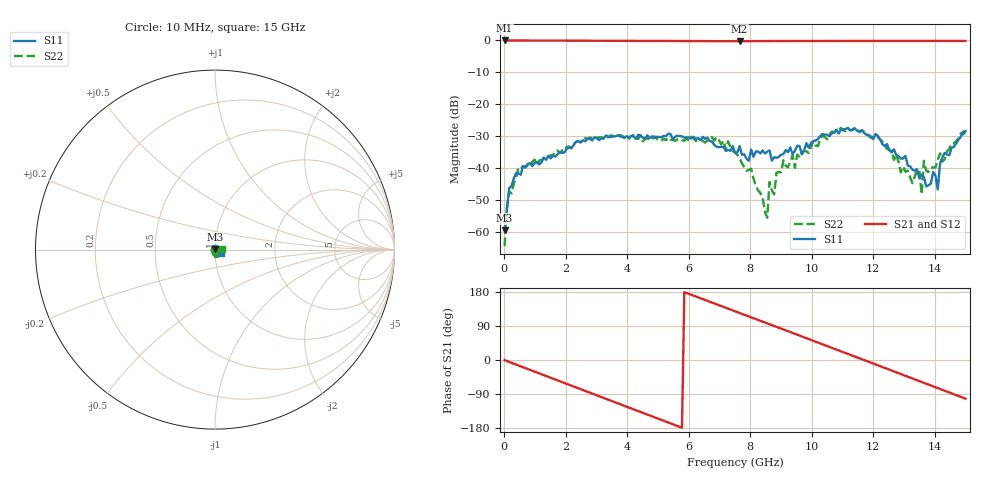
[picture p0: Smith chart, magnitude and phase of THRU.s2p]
#  HZ  S  DB  R  50.00
! Rohde & Schwarz Vector Network Analyzer
! Rohde-Schwarz,ZNB3044-4Port,1351505044101548,4.21
! Created: UTC 8/5/2026, 7:45:01 PM
! freq[Hz]  db:S11  ang:S11  db:S21  ang:S21  db:S12  ang:S12  db:S22  ang:S22
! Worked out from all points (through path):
!   201 points, 10 MHz to 15 GHz, reference 50 ohm
!   highest |S21| = 0.00 dB at 10 MHz (marker M1); lowest = -0.2 dB at 7.655 GHz (marker M2)
!   group delay of S21, straight-line fit = 85.4 ps
!   lowest |S11| = -59.6 dB at 10 MHz (marker M3), VSWR 1.00, Z = 50.1 + j0.0742 ohm
!   |S11| at or under -10 dB: start of sweep to end of sweep
!   |S22| runs from -64.6 to -27.4 dB; largest |S21 - S12| = 0.0051
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1e7  -59.61 45.1  -0.00 -0.4  -0.00 -0.3  -64.59 24.4
1.599e8  -46.34 44.9  -0.01 -5.1  -0.02 -5.1  -47.37 68.3
4.597e8  -41.70 35.1  -0.03 -14.5  -0.04 -14.5  -40.01 32.7
2.5583e9  -31.35 -6.6  -0.10 -79.3  -0.10 -79.3  -31.39 -10.4
5.03165e9  -30.27 -57.6  -0.16 -155.6  -0.16 -155.6  -31.35 -71.5
7.505e9  -35.22 -78.7  -0.23 128.5  -0.23 128.6  -35.21 -115.1
7.6549e9  -33.16 -74.6  -0.24 124.0  -0.23 124.0  -36.85 -115.8
8.5543e9  -34.87 -53.6  -0.19 96.7  -0.19 96.7  -55.66 84.7
8.62925e9  -34.53 -40.1  -0.19 94.4  -0.19 94.4  -44.42 53.8
8.77915e9  -36.67 -59.4  -0.17 89.8  -0.18 89.8  -48.36 43.7
9.07895e9  -35.71 -52.3  -0.19 80.7  -0.17 80.5  -37.62 53.7
9.4537e9  -34.62 -53.1  -0.18 69.1  -0.15 69.0  -39.98 4.8
1.00533e10  -31.62 -56.2  -0.17 50.6  -0.15 50.5  -31.66 -30.4
1.14024e10  -27.61 -80.1  -0.16 9.1  -0.14 8.9  -27.44 -82.5
1.252665e10  -34.52 -89.8  -0.15 -25.5  -0.14 -25.8  -34.36 -118.4
1.327615e10  -40.57 -53.7  -0.15 -48.7  -0.13 -48.9  -44.83 171.7
1.3501e10  -43.21 -52.9  -0.15 -55.6  -0.13 -55.8  -40.71 124.9
1.357595e10  -42.12 -66.4  -0.14 -57.9  -0.13 -58.1  -48.32 118.5
1.36509e10  -42.88 -62.3  -0.14 -60.3  -0.13 -60.4  -37.81 124.5
1.41006e10  -46.80 -11.4  -0.14 -74.2  -0.13 -74.3  -37.47 75.1
1.42505e10  -36.74 -20.8  -0.14 -78.8  -0.13 -78.9  -38.04 58.7
1.5e10  -28.49 -30.2  -0.15 -102.0  -0.14 -102.0  -28.73 2.4
